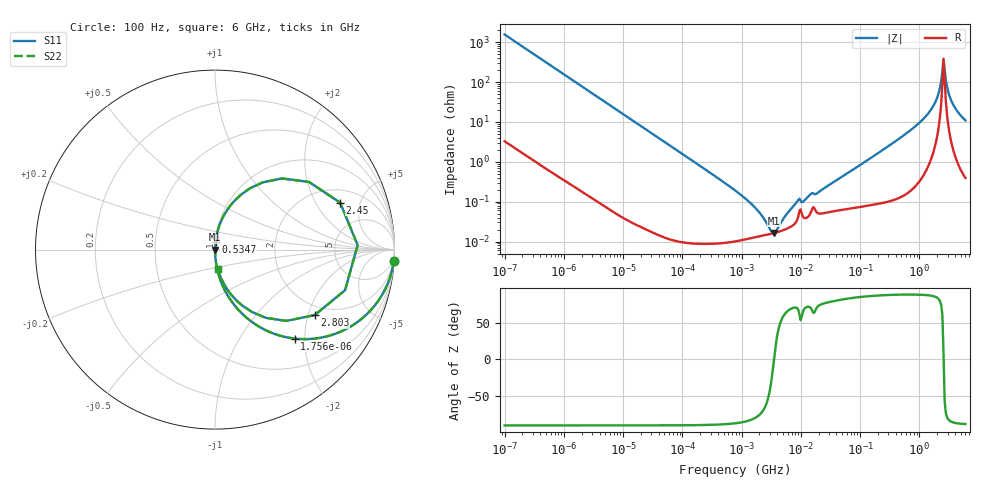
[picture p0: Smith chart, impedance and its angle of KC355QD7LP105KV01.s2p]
!Murata Part Number: KC355QD7LP105KV01
!These Parameters are Measured in Series Mode Connection
!Data Generated on Jun 19, 2026
!  o--ll--o
!Port1  Port2
!  o------o
!Operation Temp=25[degC], DC Bias Voltage=0[V]
!Freq. Start=100[Hz] Stop=6[GHz] 401[Steps]
# Hz S RI R 50
!Freq.(Hz) S11(Real) S11(Imag) S21(Real) S21(Imag) S12(Real) S12(Imag) S22(Real) S22(Imag)
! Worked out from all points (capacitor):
!   401 points, 100 Hz to 6 GHz, reference 50 ohm
!   read as one part in series: C = 1.02 uF near 109 Hz
!   lowest |Z| = 16.3 mohm at 3.55 MHz (marker M1)
!   series resonance near 3.521 MHz, so ESL is about 2 nH
!   S11 on the Smith chart (normalised r, x): 100 Hz: 1, -31; 1.756 kHz: 1.00, -1.79; 534.7 MHz: 1.00, +0.09; 2.45 GHz: 2.78, +3.27; 2.803 GHz: 1.69, -2.21; 6 GHz: 1.01, -0.22
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100  0.9958 -0.0637  0.0042 0.0637  0.0042 0.0637  0.9958 -0.0637
548  0.8905 -0.3112  0.1095 0.3112  0.1095 0.3112  0.8905 -0.3112
1756  0.4445 -0.4958  0.5555 0.4958  0.5555 0.4958  0.4445 -0.4958
2008  0.3797 -0.4842  0.6203 0.4842  0.6203 0.4842  0.3797 -0.4842
5882  0.0673 -0.2493  0.9327 0.2493  0.9327 0.2493  0.0673 -0.2493
40335  0.00167 -0.039  0.9983 0.039  0.9983 0.039  0.00167 -0.039
774597  0.000104 -0.00192  0.9999 0.00192  0.9999 0.00192  0.000104 -0.00192
1734173  0.000129 -0.000669  0.9999 0.000669  0.9999 0.000669  0.000129 -0.000669
3549919  0.000163 7.1e-06  0.9998 -7.1e-06  0.9998 -7.1e-06  0.000163 7.1e-06
8692127  0.00035 0.000944  0.9997 -0.000944  0.9997 -0.000944  0.00035 0.000944
1.137099e7  0.000391 0.000982  0.9996 -0.000982  0.9996 -0.000982  0.000391 0.000982
1.555665e7  0.000657 0.00151  0.9993 -0.00151  0.9993 -0.00151  0.000657 0.00151
3.124326e8  0.00167 0.0256  0.9983 -0.0256  0.9983 -0.0256  0.00167 0.0256
5.346885e8  0.00341 0.0449  0.9966 -0.0449  0.9966 -0.0449  0.00341 0.0449
1.094528e9  0.0152 0.1056  0.9848 -0.1056  0.9848 -0.1056  0.0152 0.1056
1.712697e9  0.0711 0.2255  0.9289 -0.2255  0.9289 -0.2255  0.0711 0.2255
2.142435e9  0.2657 0.3746  0.7343 -0.3746  0.7343 -0.3746  0.2657 0.3746
2.450438e9  0.6974 0.2615  0.3026 -0.2615  0.3026 -0.2615  0.6974 0.2615
2.802721e9  0.5559 -0.3647  0.4441 0.3647  0.4441 0.3647  0.5559 -0.3647
3.065283e9  0.2822 -0.38  0.7178 0.38  0.7178 0.38  0.2822 -0.38
3.505958e9  0.1173 -0.281  0.8827 0.281  0.8827 0.281  0.1173 -0.281
6e9  0.0155 -0.1068  0.9845 0.1068  0.9845 0.1068  0.0155 -0.1068
